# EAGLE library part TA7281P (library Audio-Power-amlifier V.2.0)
Toshiba 5,8 DUAL AUDIO POWER AMPLIEFIER
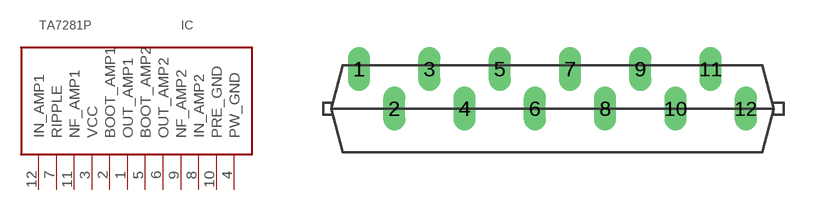
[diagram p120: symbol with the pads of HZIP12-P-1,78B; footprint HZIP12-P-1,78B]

Designator prefix IC

## TA7281P  [HZIP12-P-1,78B]
1  OUT_AMP1
2  BOOT_AMP1
3  VCC
4  PW_GND
5  BOOT_AMP2
6  OUT_AMP2
7  RIPPLE
8  IN_AMP2
9  NF_AMP2
10  PRE_GND
11  NF_AMP1
12  IN_AMP1

## Footprint HZIP12-P-1,78B (pad centres in mm)
drill 0.6 pad 1.016 long: 1 -9.779,2; 2 -8.001,0; 3 -6.223,2; 4 -4.445,0; 5 -2.667,2; 6 -0.889,0; 7 0.889,2; 8 2.667,0; 9 4.445,2; 10 6.223,0; 11 8.001,2; 12 9.779,0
